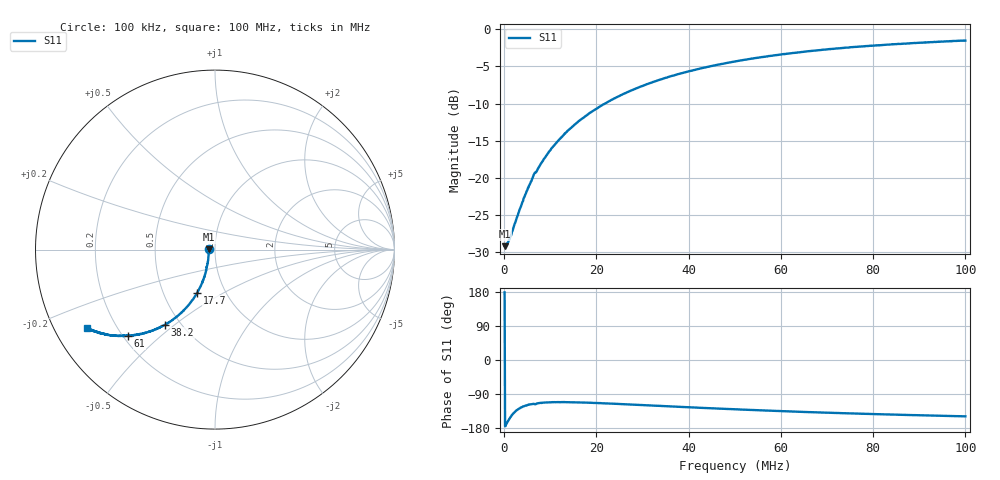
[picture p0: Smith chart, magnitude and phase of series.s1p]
# Hz S RI R 50.0
! written by SimSmith version 18.3h
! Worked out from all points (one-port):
!   1000 points, 100 kHz to 100 MHz, reference 50 ohm
!   lowest |S11| = -29.2 dB at 100 kHz (marker M1), VSWR 1.07, Z = 46.6 + j0.0847 ohm
!   |S11| at or under -10 dB: start of sweep to 21.85 MHz
!   S11 on the Smith chart (normalised r, x): 100 kHz: 0.93, +0.00; 17.7 MHz: 0.74, -0.38; 38.2 MHz: 0.41, -0.46; 61 MHz: 0.22, -0.39; 100 MHz: 0.10, -0.28
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100000  -0.0348 0.000906
400000  -0.0348 -0.00578
700000  -0.0351 -0.00988
1300000  -0.0352 -0.0189
3000000  -0.0366 -0.0432
4100000  -0.0375 -0.0591
4700000  -0.0396 -0.0677
6300000  -0.0448 -0.0924
8300000  -0.0501 -0.1193
9900000  -0.056 -0.1415
1.26e7  -0.0682 -0.1773
1.51e7  -0.083 -0.2099
1.77e7  -0.0995 -0.2414
2.1e7  -0.1243 -0.2789
2.51e7  -0.1574 -0.3204
2.77e7  -0.1805 -0.3444
3.1e7  -0.2107 -0.3718
3.76e7  -0.2734 -0.4154
3.82e7  -0.2797 -0.4187
4.34e7  -0.3297 -0.4434
5.01e7  -0.3918 -0.4634
6.1e7  -0.4847 -0.4799
6.26e7  -0.4978 -0.4807
7.04e7  -0.5552 -0.48
7.51e7  -0.587 -0.4772
8.76e7  -0.6574 -0.4588
9.57e7  -0.6975 -0.4444
1e8  -0.7153 -0.4359
